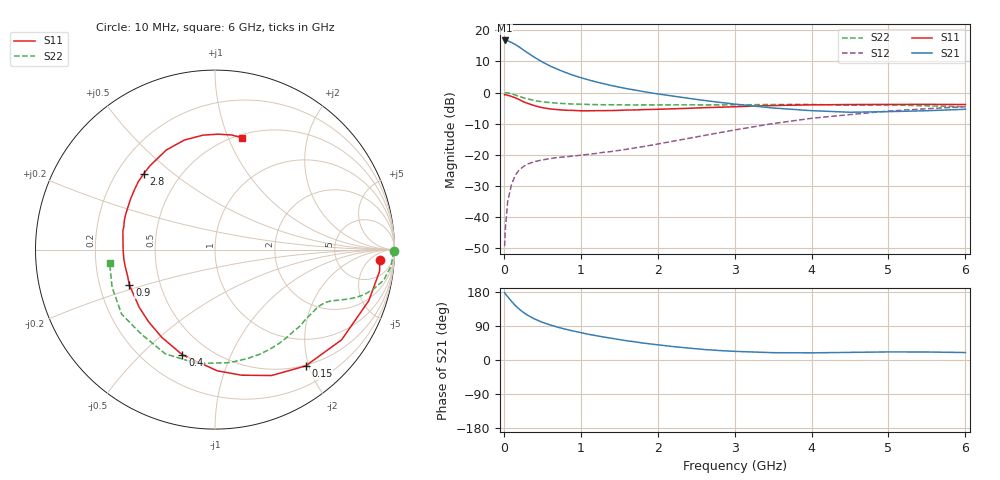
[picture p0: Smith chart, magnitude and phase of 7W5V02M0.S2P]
! Infineon Technologies  Discrete & RF Semiconductors
! BFS17W
! Si NPN RF Bipolar Junction Transistor in SOT323
! VCE = 5 V  IC = 2 mA
! Common Emitter S-Parameters:  August  1999
# GHz  S  MA  R  50
!  f  S11  S21  S12  S22
! GHz  MAG  ANG  MAG  ANG  MAG  ANG  MAG  ANG
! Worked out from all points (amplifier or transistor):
!   36 points, 10 MHz to 6 GHz, reference 50 ohm
!   highest |S21| = 16.7 dB at 10 MHz (marker M1)
!   |S21| within 3 dB of that: start of sweep to 252.2 MHz
!   unconditionally stable (mu >= 1): 834.7 MHz to 3.059 GHz; 4.133 GHz to end of sweep
!   at 250 MHz: K = 0.35, MSG = 18.8 dB, |S12| = -23.9 dB
!   at 1.4 GHz: K = 1.28, MAG = 7.4 dB, |S12| = -19.0 dB
!   at 6 GHz: K = 1.08, MAG = -2.2 dB, |S12| = -4.6 dB
!   S11 on the Smith chart (normalised r, x): 10 MHz: 15, -12; 150 MHz: 0.49, -1.95; 400 MHz: 0.36, -0.67; 900 MHz: 0.33, -0.18; 2.8 GHz: 0.31, +0.40; 6 GHz: 0.53, +1.12
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0.01  0.9203 -3.6  6.861 178.0  0.0034 86.8  0.9993 -0.6
0.02  0.9248 -7.5  6.816 174.7  0.0066 87.7  0.9911 -2.2
0.05  0.9029 -18.4  6.75 166.8  0.0178 81.3  0.9848 -5.5
0.1  0.8661 -35.5  6.354 154.8  0.0334 71.6  0.955 -10.3
0.15  0.8214 -52.1  5.908 143.5  0.0471 62.8  0.9087 -14.1
0.2  0.7692 -65.8  5.389 134.2  0.0572 57.2  0.8669 -16.9
0.25  0.7155 -78.0  4.879 126.1  0.0639 52.0  0.8255 -18.9
0.3  0.6756 -88.9  4.411 119.3  0.0704 48.4  0.7936 -20.3
0.4  0.6138 -107.2  3.668 108.1  0.0778 44.0  0.7426 -22.3
0.5  0.5716 -121.3  3.101 99.6  0.0825 41.4  0.7098 -23.7
0.6  0.546 -132.8  2.671 92.6  0.0869 40.7  0.6884 -25.1
0.7  0.531 -142.5  2.358 86.6  0.0905 41.0  0.6733 -26.6
0.9  0.5163 -157.4  1.896 76.6  0.0952 42.9  0.6534 -30.0
1.1  0.5092 -169.4  1.597 67.9  0.1017 46.1  0.6437 -34.0
1.3  0.5118 -179.5  1.383 60.6  0.1097 49.7  0.6366 -38.5
1.6  0.5236 168.6  1.152 50.7  0.1228 55.1  0.6317 -45.5
2.2  0.5474 149.7  0.875 35.4  0.1652 63.9  0.6335 -61.2
2.8  0.5799 133.2  0.696 25.0  0.2258 66.8  0.6331 -78.3
3.5  0.6177 116.1  0.564 19.3  0.3173 64.0  0.6419 -98.8
4.5  0.6411 96.0  0.482 20.1  0.4424 52.1  0.6246 -131.0
5.5  0.6452 81.8  0.51 21.1  0.5489 38.9  0.6106 -160.0
6  0.6413 76.5  0.538 19.7  0.5903 32.5  0.5918 -172.8
